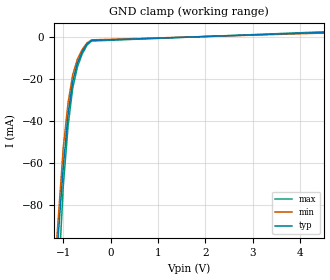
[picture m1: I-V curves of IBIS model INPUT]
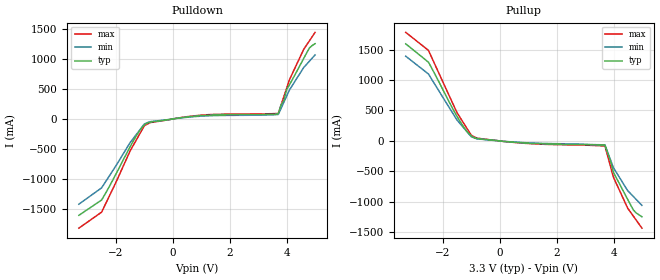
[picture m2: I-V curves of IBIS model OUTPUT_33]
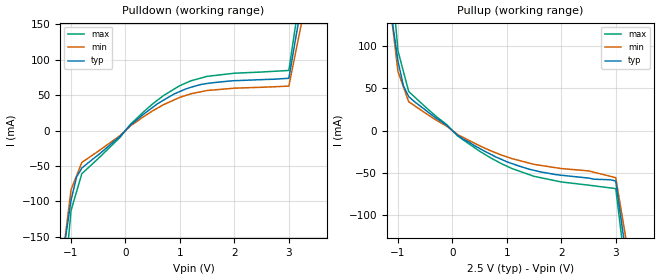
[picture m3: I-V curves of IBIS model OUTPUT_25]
|   PERICOM SEMICONDUCTOR CORP
|   IBIS Model of PI6C49X0204A
|   Product Family: PI6C49Xxxx
|   SOIC (W) 8-pin Package
[IBIS Ver] 3.2
[Comment char] |_char
[File Name] pi6c49x0204a.ibs
[File Rev] 2.0
[Source] File originated at Pericom Semiconductor Corp.
[Date] 03/16/15
[Disclaimer] (C) Copyright PERICOM Semiconductor Corporation
   All rights reserved
  Pericom Semiconductor Corporation hereby grants the user of
  this IBIS model a non-exclusive, nontransferable license to
  use this IBIS model under the following terms.
  This IBIS model is provided on an "AS IS" basis and Pericom
  makes absolutely no warranty with respect to the information
  contained herein. PERICOM DISCLAIMS AND CUSTOMER WAIVES ALL
  WARRANTIES, EXPRESSED OR IMPLIED, INCLUDING WARRANTIES OF
  MERCHANTABILITY OR FITNESS FOR A PARTICULAR PURPOSE. The
  entire risk as to quality and performance is with the customer.
  Accordingly, in no event shall the company be liable for any
  damages, whether in contract or tort, including any lost
  profits or other incidental, consequential, exemplary, or
  punitive damages arising out of the use or application of the
  IBIS model provided in this package. Further, Pericom reserves
  the right to make changes without notice to any product herein
  to improve reliability, function, or design. Pericom does not
  convey any license under patent rights or any other intellectual
  property rights, including those of third parties.
  The user is granted this license only to use the IBIS model
  and is not granted rights to sell, load, rent, lease or license
  the IBIS model in whole or in part, or in modified form to anyone
  other than user. User may modify the IBIS model to suit its specific
  application but rights to derivative works and such modifications
  shall belong to Pericom.
  Pericom is not obligated to provide maintenance or support
  for the licensed IBIS model.
  Contact Pericom at ATTN: APPLICATION ENGINEERING / IBIS MODELS
  3545 North First Street, San Jose, CA 95134
[Component] pi6c49x0204a
[Manufacturer] Pericom Semiconductor Corp.
[Package]
| variable   typ   min  max
R_pkg   0.52715ohm  0.474435	0.579865
L_pkg   1.17050nH   1.01345nH	1.22755nH
C_pkg   0.29280pF   0.26352pF	0.32208pF
[Pin]   Signal_Name   Model_Name   R_pin   L_pin   C_pin
1   CLK   INPUT   0.05164   1.483nH   0.3562pF
2   Q1   OUTPUT   0.05379   1.258nH   0.2294pF
3   Q2   OUTPUT   0.05379   1.258nH   0.2294pF
4   Q3   OUTPUT   0.05379   1.258nH   0.2294pF
5   Q4   OUTPUT   0.05379   1.258nH   0.2294pF
6   GND   GND   0.05379   1.458nH   0.2294pF
7   VDD   POWER   0.05379   1.458nH   0.2294pF
8   OE   INPUT   0.05164   1.483nH   0.3562pF
| OUTPUT model selection
[Model Selector]   OUTPUT
OUTPUT_33   3.3 volt VDD
OUTPUT_25   2.5 volt VDD
OUTPUT_18   1.8 volt VDD
OUTPUT_15   1.5 volt VDD
| Models and submodels in the file (5): INPUT (Input), OUTPUT_33 (Output), OUTPUT_25 (Output), OUTPUT_18 (Output), OUTPUT_15 (Output)
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|   Model INPUT
[Model] INPUT
Model_type Input
Vinl = 400mV
Vinh = 3.0V
| variable   typ   min   max
C_comp   2.000pF   1.8pF	2.2pF
[Voltage Range]   3.300V   3.0	 3.6
[POWER Clamp Reference]   2.500V   NA   NA
[GND Clamp Reference]   0.000V   0	 0
[Pullup Reference]   3.300V   3.3	 3.3
[Pulldown Reference]   0.000V   NA   NA
[Temperature Range]   25.00   85.00   -45.000
[GND Clamp]
| Voltage   I(typ)   I(min)   I(max)
-2.501V   -689.3mA   -585.9mA   -792.7mA
-1.202V   -128.3mA   NA         NA
-1.1V     -92.86mA   NA         NA
-999.3mV  -61.6mA    -52.36mA   -70.84mA
-898.2mV  -36.82mA   -31.3mA    -42.34mA
-802mV    -21.38mA   -18.17mA   -24.59mA
-700.9mV  -12.48mA   -10.61mA   -14.35mA
-599.7mV  -7.15mA    -6.077mA   -8.223mA
-498.6mV  -3.5mA     -2.975mA   -4.025mA
-402.7mV  -1.81mA    -1.538mA   -2.082mA
4.999V    2.38mA     2.023mA    2.737mA
[POWER Clamp]   |Note: Vtable = Vcc - Voutput
| Voltage   I(typ)   I(min)   I(max)
-2.501V   0A         0A         0A
0V        0A         0A         0A
|   Model OUTPUT_33
[Model] OUTPUT_33
Model_type Output
Vref = 0.0000V
Rref = 50ohms
Vmeas = 1.650V
| variable   typ   min   max
C_comp   2.000pF   1.8pF	2.2pF
[Voltage Range]   3.300V   3.0	 3.6
[POWER Clamp Reference]   3.300V   NA   NA
[GND Clamp Reference]   0.000V   0	 0
[Pullup Reference]   3.300V   3.0	 3.6
[Pulldown Reference]   0.000V   NA   NA
[Temperature Range]   25.00   85.00   -45.000
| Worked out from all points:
|   slope of the pulldown table from 0 to 0.495 V, typ, clamps not added: 15.3 ohm
|   slope of the pullup table from 0 to 0.495 V, typ, clamps not added: 23.5 ohm
[Pulldown]
| Voltage   I(typ)   I(min)  I(max)
-3.3V     -1.601A    -1.416A    -1.813A
-2.501V   -1.346A    -1.144A    -1.548A
-1.5V     -461.9mA   -392.6mA   -531.2mA
-999.3mV  -97.83mA   -83.16mA   -112.5mA
999.4mV   55.02mA    46.77mA    63.27mA
3.708V    85.7mA     74.84mA    93.55mA
3.901V    306mA      NA         NA
3.997V    482.3mA    NA         NA
4.099V    566.4mA    481.4mA    651.3mA
4.599V    1.005A     854.5mA    1.156A
4.802V    1.181A     NA         NA
4.999V    1.25A      1.063A     1.438A
[Pullup]   |Note: Vtable = Vcc - Voutput
| Voltage   I(typ)   I(min)   I(max)
-3.3V     1.593A     1.39A      1.781A
-2.501V   1.292A     1.098A     1.485A
-1.5V     403.8mA    343.2mA    464.4mA
-999.4mV  82.22mA    69.89mA    94.55mA
-802mV    40.18mA    34.15mA    46.21mA
700.9mV   -28.06mA   -23.85mA   -32.27mA
3.699V    -68.29mA   -65.3mA    -82.28mA
3.901V    -336mA     NA         NA
3.997V    -517.9mA   -440.2mA   -595.6mA
4.498V    -959.4mA   -815.5mA   -1.103A
4.7V      -1.135A    NA         NA
4.999V    -1.244A    -1.058A    -1.431A
[Ramp]
| variable   typ   min   max
dV/dt_r   2.5V/941.0p   2.5V/1041.0p   2.5V/841.0p
dV/dt_f   2.5V/806.0p   2.5V/1006.0p   2.5V/706.0p
R_load = 50ohms
|   Model OUTPUT_25
[Model] OUTPUT_25
Model_type Output
Vref = 0.0000V
Rref = 50ohms
Vmeas = 1.250V
| variable   typ   min   max
C_comp   2.000pF   1.8pF	2.2pF
[Voltage Range]   2.500V   2.375	 2.625
[POWER Clamp Reference]   2.500V   NA   NA
[GND Clamp Reference]   0.000V   0	 0
[Pullup Reference]   2.500V   2.375	 2.625
[Pulldown Reference]   0.000V   NA   NA
[Temperature Range]   25.00   85.00   -45.000
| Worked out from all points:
|   slope of the pulldown table from 0 to 0.375 V, typ, clamps not added: 14.8 ohm
|   slope of the pullup table from 0 to 0.375 V, typ, clamps not added: 22.6 ohm
[Pulldown]
| Voltage   I(typ)   I(min)  I(max)
-2.501V   -1.346A    -1.144A    -1.548A
-1.1V     -151.1mA   NA         NA
-999.3mV  -97.83mA   -83.16mA   -112.5mA
-898.2mV  -65.44mA   NA         NA
-802mV    -52.94mA   -45mA      -60.88mA
-99.45mV  -8.35mA    -7.097mA   -9.602mA
99.45mV   8.25mA     7.012mA    9.487mA
700.9mV   42.95mA    36.51mA    49.39mA
999.4mV   55.02mA    46.77mA    63.27mA
1.5V      66.36mA    56.41mA    76.31mA
3.002V    73.6mA     62.56mA    84.64mA
4.099V    566.4mA    481.4mA    651.3mA
[Pullup]   |Note: Vtable = Vcc - Voutput
| Voltage   I(typ)   I(min)   I(max)
-2.501V   1.292A     1.098A     1.485A
-1.1V     128.3mA    NA         NA
-999.4mV  82.22mA    69.89mA    94.55mA
-898.2mV  52.83mA    NA         NA
-802mV    40.18mA    34.15mA    46.21mA
-99.45mV  5.88mA     4.998mA    6.762mA
99.44mV   -5.76mA    -4.896mA   -6.624mA
898.2mV   -34.05mA   -28.94mA   -39.16mA
1.5V      -47.14mA   -40.07mA   -54.21mA
2.501V    -56.24mA   -47.8mA    -64.68mA
3.002V    -59.8mA    -55.83mA   -68.77mA
3.997V    -517.9mA   -440.2mA   -595.6mA
[Ramp]
| variable   typ   min   max
dV/dt_r   1.9V/941.0p   1.9V/1041.0p   1.9V/841.0p
dV/dt_f   1.9V/806.0p   1.9V/1006.0p   1.9V/706.0p
R_load = 50ohms
